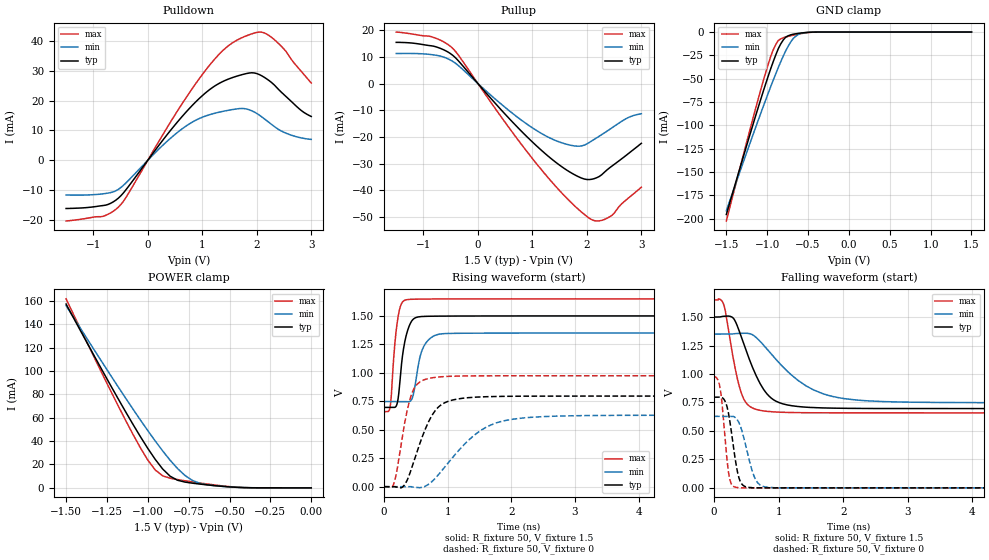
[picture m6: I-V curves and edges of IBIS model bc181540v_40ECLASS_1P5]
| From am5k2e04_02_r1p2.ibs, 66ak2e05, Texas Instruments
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|   Model Cell bc181540v_40ECLASS_1P5
|bc181540v_40ECLASS_1P5
[Model]   bc181540v_40ECLASS_1P5
Model_type   I/O
Polarity   Non-Inverting
Enable   Active-Low
Vinl =  0.525
Vinh =  0.975
Cref =  15.0000pF
Rref =  100.0000M
Vref =  0V
Vmeas =  0.75
C_comp   1.17072p   0.570099p   1.17447p
[Model Spec]
Vinl   0.525   0.4725   0.5775
Vinh   0.975   0.8775   1.0725
[Temperature Range]   25   125   -40
[Voltage Range]   1.5   1.35   1.65
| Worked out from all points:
|   slope of the pulldown table from 0 to 0.225 V, typ, clamps not added: 40.7 ohm
|   slope of the pullup table from 0 to 0.225 V, typ, clamps not added: 42.7 ohm
|   GND clamp passes 1 mA (typ) near -0.58 V on its own axis
|   POWER clamp passes 1 mA (typ) near -0.52 V on its own axis
|   rising waveform, R_fixture 50, V_fixture 1.5: 20-80 % time 114ps typ, 140ps min, 88.3ps max; typ from 0.696 V to 1.5 V
|   rising waveform, R_fixture 50, V_fixture 0: 20-80 % time 333ps typ, 657ps min, 196ps max; typ from 0 V to 0.796 V
|   falling waveform, R_fixture 50, V_fixture 1.5: 20-80 % time 363ps typ, 710ps min, 204ps max; typ from 1.5 V to 0.696 V
|   falling waveform, R_fixture 50, V_fixture 0: 20-80 % time 126ps typ, 173ps min, 94.4ps max; typ from 0.796 V to 0 V
[POWER_clamp]
|   voltage   I(typ)   I(min)   I(max)
-1.5V     157.2mA    155.9mA    161.7mA
-1.273V   98.95mA    106mA      95.87mA
-1.091V   54.38mA    67.4mA     45.82mA
-1V       33.74mA    48.95mA    23.8mA
-954.5mV  24.35mA    40.1mA     15.29mA
-909.1mV  16.14mA    31.61mA    10.28mA
-863.6mV  9.975mA    23.68mA    8.252mA
-818.2mV  6.508mA    16.53mA    7.086mA
-727.3mV  4mA        6.353mA    5.092mA
-681.8mV  3.231mA    3.88mA     4.159mA
-409.1mV  177.3uA    258.7uA    224.6uA
0V        677pA      15.94nA    186.8pA
[Pulldown]
|   voltage   I(typ)   I(min)   I(max)
-1.5V     -16.18mA   -11.66mA   -20.38mA
-818.2mV  -15.18mA   -11.25mA   -18.79mA
-500mV    -12.01mA   -9.214mA   -14.96mA
272.7mV   6.67mA     4.988mA    8.497mA
727.3mV   16.67mA    11.78mA    21.68mA
1.273V    25.41mA    15.97mA    34.86mA
1.636V    28.23mA    17.24mA    40.29mA
1.955V    29.29mA    16.18mA    42.68mA
2.182V    27.31mA    13.3mA     42.34mA
2.545V    21.24mA    9.012mA    36.3mA
2.818V    16.68mA    7.5mA      29.79mA
3V        14.69mA    6.98mA     25.92mA
[Pullup]
|   voltage   I(typ)   I(min)   I(max)
-1.5V     15.42mA    11.25mA    19.29mA
-863.6mV  14.15mA    10.86mA    17.6mA
-454.5mV  10.44mA    8.203mA    13.01mA
545.5mV   -12.48mA   -9.696mA   -15.83mA
1.136V    -24.46mA   -18.34mA   -31.54mA
1.727V    -33.62mA   -23.21mA   -44.88mA
1.909V    -35.45mA   -23.32mA   -48.26mA
2.045V    -35.95mA   -22.05mA   -50.44mA
2.227V    -34.79mA   -19.71mA   -51.42mA
2.409V    -31.68mA   -17.28mA   -50.01mA
2.773V    -26.05mA   -12.61mA   -42.7mA
3V        -22.38mA   -11.31mA   -38.83mA
[GND_clamp]
|   voltage   I(typ)   I(min)   I(max)
-1.5V     -195.7mA   -191.7mA   -202.6mA
-1.227V   -114.7mA   -123.3mA   -110.1mA
-1.045V   -62.85mA   -79.19mA   -51.48mA
-954.5mV  -38.7mA    -58mA      -25.52mA
-893.9mV  -24.32mA   -44.5mA    -13.19mA
-863.6mV  -17.74mA   -37.93mA   -9.007mA
-772.7mV  -5.381mA   -20.03mA   -5.301mA
-681.8mV  -2.343mA   -6.948mA   -3.394mA
-621.2mV  -1.47mA    -2.783mA   -2.285mA
-560.6mV  -800.4uA   -1.037mA   -1.331mA
-348.5mV  -9.367uA   -19.45uA   -12.08uA
1.5V      677pA      908.2nA    87.75pA
[Ramp]
| variable   typ   min   max
dV/dt_f   0.487548/0.36543382n   0.365916/0.71447287n   0.600714/0.20512877n
dV/dt_r  0.4837218/0.33565985n 0.38231568/0.66274953n 0.58878498/0.19650698n
R_load = 50
[Rising Waveform]
R_fixture = 50
V_fixture = 1.5
V_fixture_min = 1.35
V_fixture_max = 1.65
|   time   V(typ)   V(min)   V(max)
0s        696.1mV    747.8mV    659.1mV
103.1ps   696.2mV    747.8mV    722.3mV
158.5ps   695.6mV    747.8mV    1.173V
206.5ps   727.6mV    747.8mV    1.435V
296.2ps   1.171V     747.9mV    1.626V
380.5ps   1.388V     746mV      1.645V
460.5ps   1.472V     807.5mV    1.647V
630.1ps   1.496V     1.238V     1.649V
924.9ps   1.499V     1.344V     1.65V
16.75ns   1.5V       1.35V      1.65V
[Rising Waveform]
R_fixture = 50
V_fixture = 0
V_fixture_min = 0
V_fixture_max = 0
|   time   V(typ)   V(min)   V(max)
0s        0V         0V         0V
162ps     0V         0V         39.35mV
318.8ps   12.83mV    0V         538.4mV
394.6ps   97.77mV    0V         739.6mV
470.7ps   224.4mV    -4.385mV   859.8mV
686.6ps   554.2mV    15.86mV    948.5mV
844.6ps   693.8mV    98.49mV    962.9mV
1.522ns   788.6mV    495.3mV    973.9mV
2.302ns   795.3mV    609.1mV    974.5mV
16.71ns   795.9mV    627.8mV    974.5mV
[Falling Waveform]
R_fixture = 50
V_fixture = 1.5
V_fixture_min = 1.35
V_fixture_max = 1.65
|   time   V(typ)   V(min)   V(max)
0s        1.5V       1.35V      1.65V
150.1ps   1.507V     1.35V      1.609V
310.5ps   1.481V     1.353V     1.096V
459.7ps   1.264V     1.358V     780.4mV
626.6ps   1.016V     1.332V     693.8mV
801.1ps   838mV      1.231V     672.8mV
1.051ns   739.7mV    1.071V     663.6mV
1.54ns    704.8mV    860.3mV    659.2mV
2.378ns   697mV      764mV      658.5mV
16.75ns   696.1mV    747.8mV    658.4mV
[Falling Waveform]
R_fixture = 50
V_fixture = 0
V_fixture_min = 0
V_fixture_max = 0
|   time   V(typ)   V(min)   V(max)
0s        795.9mV    627.8mV    974.5mV
96.3ps    797mV      627.8mV    867.2mV
198ps     718.9mV    627.8mV    261.8mV
232.8ps   624.9mV    627.7mV    103.9mV
263.5ps   509.9mV    628.4mV    38.81mV
384.6ps   88.98mV    572.7mV    0V
459.6ps   17.63mV    442.2mV    0V
650ps     0V         65.3mV     0V
941.2ps   0V         0V         0V
16.71ns   0V         0V         0V
